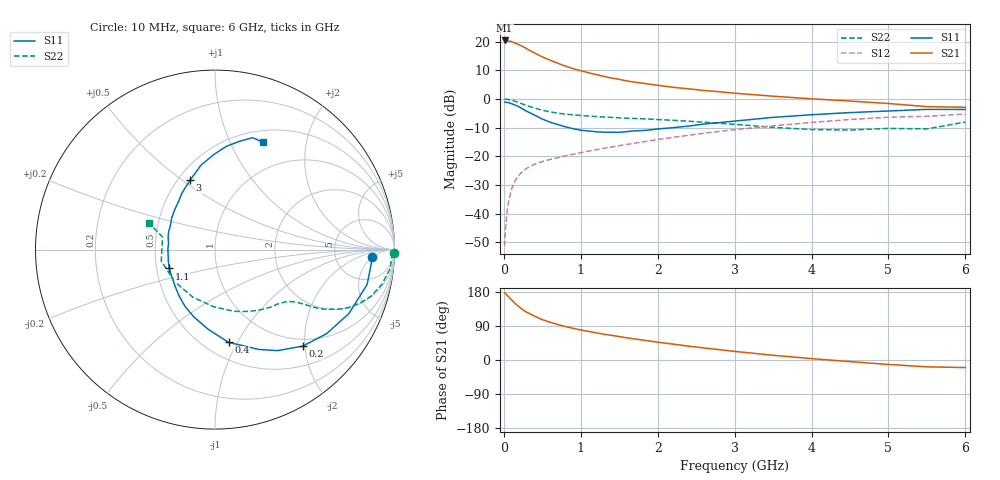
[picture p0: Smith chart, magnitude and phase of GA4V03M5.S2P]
! Infineon Technologies  Discrete & RF Semiconductors
! BF775
! Si NPN RF Bipolar Junction Transistor in SOT23
! VCE = 4 V  IC = 3.5 mA
! Common Emitter S-Parameters:  May  1996
# GHz  S  MA  R  50
!  f  S11  S21  S12  S22
! GHz  MAG  ANG  MAG  ANG  MAG  ANG  MAG  ANG
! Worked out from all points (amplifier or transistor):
!   36 points, 10 MHz to 6 GHz, reference 50 ohm
!   highest |S21| = 20.4 dB at 10 MHz (marker M1)
!   |S21| within 3 dB of that: start of sweep to 304.1 MHz
!   unconditionally stable (mu >= 1): 939.6 MHz to 3.447 GHz
!   at 250 MHz: K = 0.39, MSG = 21.7 dB, |S12| = -25.1 dB
!   at 1.4 GHz: K = 1.13, MAG = 9.9 dB, |S12| = -16.8 dB
!   at 6 GHz: K = 0.96, MSG = 1.2 dB, |S12| = -5.3 dB
!   S11 on the Smith chart (normalised r, x): 10 MHz: 14, -5; 200 MHz: 0.86, -1.95; 400 MHz: 0.65, -0.92; 1.1 GHz: 0.58, -0.13; 3 GHz: 0.57, +0.54; 6 GHz: 0.64, +1.34
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0.01  0.8774 -2.6  10.48 177.9  0.0027 88.2  0.9952 -1.2
0.02  0.8742 -5.1  10.37 175.4  0.0053 89.4  0.9848 -2.5
0.05  0.8697 -12.9  10.29 169.2  0.0137 82.5  0.9821 -6.1
0.1  0.8265 -25.6  10.04 158.8  0.0267 75.8  0.9504 -11.7
0.15  0.7785 -37.0  9.381 148.5  0.0381 70.2  0.9073 -16.6
0.2  0.7263 -47.8  8.775 140.2  0.0473 65.5  0.8606 -20.3
0.25  0.6623 -58.2  8.16 132.2  0.0556 61.4  0.8092 -23.6
0.3  0.6076 -66.3  7.471 125.7  0.0618 59.0  0.7637 -25.8
0.4  0.522 -81.7  6.329 115.8  0.0726 54.9  0.6931 -28.6
0.5  0.4458 -94.9  5.412 106.5  0.0807 53.1  0.6373 -30.3
0.6  0.393 -107.5  4.746 99.6  0.0878 52.0  0.5955 -31.2
0.7  0.3577 -117.9  4.195 93.7  0.0944 52.1  0.5659 -32.0
0.9  0.3028 -137.0  3.372 83.6  0.1083 52.0  0.5273 -33.5
1.1  0.2759 -157.7  2.87 75.5  0.1229 53.0  0.5035 -35.3
1.3  0.263 -173.1  2.473 68.2  0.1377 53.6  0.4835 -37.2
1.6  0.2694 165.7  2.062 58.5  0.1611 53.7  0.4609 -41.2
2.2  0.3155 135.5  1.596 41.8  0.2135 52.0  0.424 -51.9
3  0.4108 109.7  1.259 22.7  0.2909 45.9  0.3609 -72.4
3.5  0.477 99.4  1.117 12.5  0.3394 40.8  0.3199 -90.7
4.5  0.5782 83.8  0.919 -4.3  0.4378 28.3  0.2872 -141.9
5.5  0.6576 71.5  0.734 -18.0  0.498 13.0  0.3007 166.5
6  0.6556 66.0  0.716 -20.0  0.5445 8.8  0.3951 158.2
